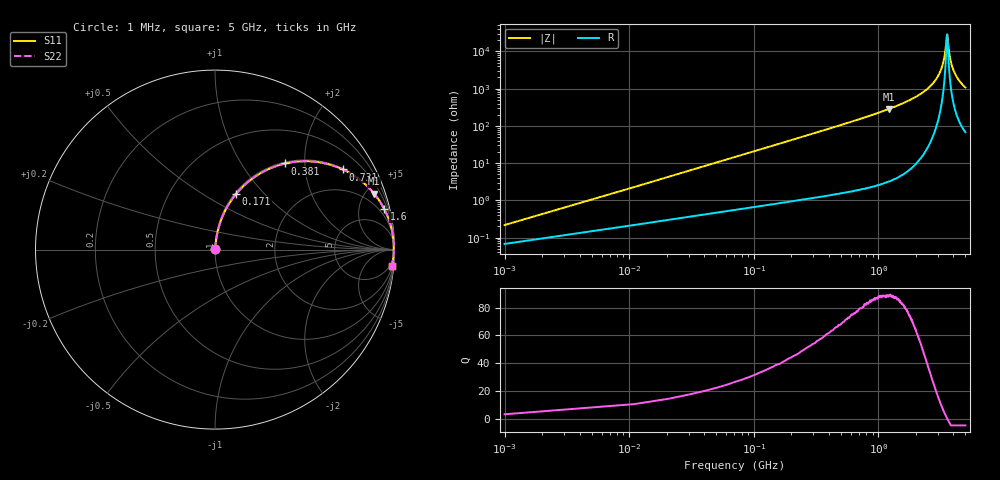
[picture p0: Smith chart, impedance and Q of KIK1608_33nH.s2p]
!version-2
!date-01.2022
!Series
# MHz S RI R 50
!Freq ReS11 ImS11 ReS21 ImS21 ReS12 ImS12 ReS22 ImS22
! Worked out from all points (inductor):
!   501 points, 1 MHz to 5 GHz, reference 50 ohm
!   read as one part in series: L = 33 nH near 21 MHz
!   highest Q = 88.8 at 1.21 GHz (marker M1), where L = 37.3 nH
!   self-resonance near 3.56 GHz
!   S11 on the Smith chart (normalised r, x): 1 MHz: 1.00, +0.00; 171 MHz: 1.02, +0.71; 381 MHz: 1.03, +1.60; 731 MHz: 1.04, +3.16; 1.6 GHz: 1.10, +8.31; 5 GHz: 2, -21
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1  0.000666 0.00207  0.9993 -0.00207  0.9993 -0.00207  0.000666 0.00207
31  0.00774 0.0635  0.9923 -0.0635  0.9923 -0.0635  0.00774 0.0635
51  0.0156 0.1036  0.9844 -0.1036  0.9844 -0.1036  0.0156 0.1036
101  0.0479 0.1982  0.9521 -0.1982  0.9521 -0.1982  0.0479 0.1982
171  0.1181 0.3107  0.8819 -0.3107  0.8819 -0.3107  0.1181 0.3107
381  0.3915 0.4799  0.6085 -0.4799  0.6085 -0.4799  0.3915 0.4799
731  0.7122 0.4465  0.2878 -0.4465  0.2878 -0.4465  0.7122 0.4465
841  0.7705 0.4146  0.2295 -0.4146  0.2295 -0.4146  0.7705 0.4146
1210  0.8868 0.3112  0.1132 -0.3112  0.1132 -0.3112  0.8868 0.3112
1600  0.9428 0.2262  0.0572 -0.2262  0.0572 -0.2262  0.9428 0.2262
1670  0.9492 0.2133  0.0508 -0.2133  0.0508 -0.2133  0.9492 0.2133
2510  0.9882 0.0956  0.0118 -0.0956  0.0118 -0.0956  0.9882 0.0956
3030  0.9951 0.044  0.00486 -0.044  0.00486 -0.044  0.9951 0.044
3340  0.9965 0.0178  0.00353 -0.0178  0.00353 -0.0178  0.9965 0.0178
3440  0.9966 0.00985  0.00343 -0.00985  0.00343 -0.00985  0.9966 0.00985
3540  0.9965 0.00217  0.00345 -0.00217  0.00345 -0.00217  0.9965 0.00217
3570  0.9965 -9.63e-05  0.00349 9.63e-05  0.00349 9.63e-05  0.9965 -9.63e-05
3700  0.9963 -0.00968  0.00375 0.00968  0.00375 0.00968  0.9963 -0.00968
3800  0.9959 -0.0168  0.00407 0.0168  0.00407 0.0168  0.9959 -0.0168
3960  0.9952 -0.0279  0.0048 0.0279  0.0048 0.0279  0.9952 -0.0279
4170  0.9939 -0.0418  0.0061 0.0418  0.0061 0.0418  0.9939 -0.0418
5000  0.9858 -0.0909  0.0142 0.0909  0.0142 0.0909  0.9858 -0.0909
